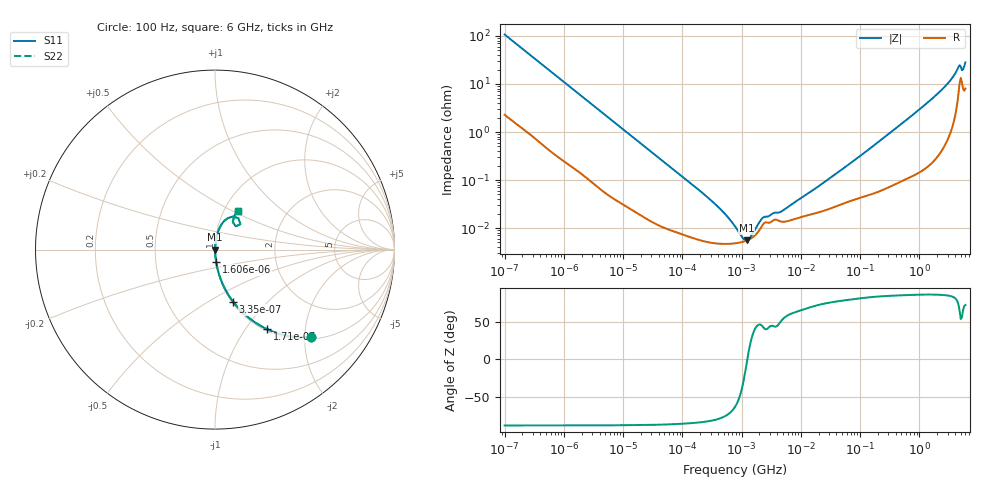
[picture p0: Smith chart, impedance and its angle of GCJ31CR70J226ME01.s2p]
!Murata Part Number: GCJ31CR70J226ME01
!These Parameters are Measured in Series Mode Connection
!Data Generated on Mar 13, 2026
!  o--ll--o
!Port1  Port2
!  o------o
!Operation Temp=25[degC], DC Bias Voltage=0[V]
!Freq. Start=100[Hz] Stop=6[GHz] 401[Steps]
# Hz S RI R 50
!Freq.(Hz) S11(Real) S11(Imag) S21(Real) S21(Imag) S12(Real) S12(Imag) S22(Real) S22(Imag)
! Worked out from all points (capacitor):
!   401 points, 100 Hz to 6 GHz, reference 50 ohm
!   read as one part in series: C = 14.7 uF near 109 Hz
!   lowest |Z| = 5.52 mohm at 1.212 MHz (marker M1)
!   series resonance near 1.249 MHz, so ESL is about 1.1 nH
!   S11 on the Smith chart (normalised r, x): 100 Hz: 1.05, -2.15; 171 Hz: 1.03, -1.26; 335 Hz: 1.01, -0.65; 1.606 kHz: 1.00, -0.14; 6 GHz: 1.16, +0.54
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100  0.5353 -0.4882  0.4647 0.4882  0.4647 0.4882  0.5353 -0.4882
171  0.2898 -0.4429  0.7102 0.4429  0.7102 0.4429  0.2898 -0.4429
335  0.1013 -0.291  0.8987 0.291  0.8987 0.291  0.1013 -0.291
717  0.0262 -0.1493  0.9738 0.1493  0.9738 0.1493  0.0262 -0.1493
1606  0.00641 -0.0689  0.9936 0.0689  0.9936 0.0689  0.00641 -0.0689
2008  0.00441 -0.0554  0.9956 0.0554  0.9956 0.0554  0.00441 -0.0554
40335  0.000121 -0.0029  0.9999 0.0029  0.9999 0.0029  0.000121 -0.0029
316350  4.91e-05 -0.000359  1 0.000359  1 0.000359  4.91e-05 -0.000359
517687  4.67e-05 -0.000195  1 0.000195  1 0.000195  4.67e-05 -0.000195
774597  4.8e-05 -9.74e-05  1 9.74e-05  1 9.74e-05  4.8e-05 -9.74e-05
885955  4.92e-05 -6.89e-05  1 6.89e-05  1 6.89e-05  4.92e-05 -6.89e-05
1212075  5.49e-05 -6e-06  0.9999 6e-06  0.9999 6e-06  5.49e-05 -6e-06
1658239  6.9e-05 5.78e-05  0.9999 -5.78e-05  0.9999 -5.78e-05  6.9e-05 5.78e-05
2372521  0.000125 0.000114  0.9999 -0.000114  0.9999 -0.000114  0.000125 0.000114
4643984  0.000136 0.000172  0.9999 -0.000172  0.9999 -0.000172  0.000136 0.000172
1.555665e7  0.000195 0.000567  0.9998 -0.000567  0.9998 -0.000567  0.000195 0.000567
3.124326e8  0.000802 0.00933  0.9992 -0.00933  0.9992 -0.00933  0.000802 0.00933
1.369159e9  0.0035 0.0404  0.9965 -0.0404  0.9965 -0.0404  0.0035 0.0404
2.931063e9  0.0158 0.0959  0.9842 -0.0959  0.9842 -0.0959  0.0158 0.0959
4.385646e9  0.0723 0.1757  0.9277 -0.1757  0.9277 -0.1757  0.0723 0.1757
5.245841e9  0.1156 0.1295  0.8844 -0.1295  0.8844 -0.1295  0.1156 0.1295
6e9  0.1287 0.2174  0.8713 -0.2174  0.8713 -0.2174  0.1287 0.2174
